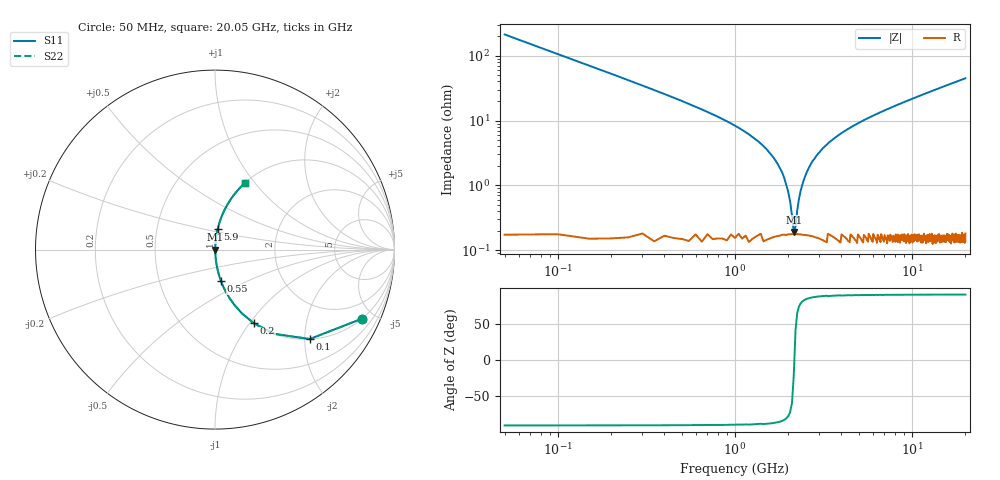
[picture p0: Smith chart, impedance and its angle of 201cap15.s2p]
! AVX Thin Film Operation		Date: May 2007
! Description: Accu-P® Series, Thin Film, SMD, RF Capacitor
! Part Number: 0201ZK150FBS
! 50 MHz  -  20.05 GHz
! Serial Measurements
# MHZ S MA R 50
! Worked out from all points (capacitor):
!   401 points, 50 MHz to 20.05 GHz, reference 50 ohm
!   read as one part in series: C = 15 pF near 150 MHz
!   lowest |Z| = 192 mohm at 2.15 GHz (marker M1)
!   series resonance near 2.166 GHz, so ESL is about 360 pH
!   S11 on the Smith chart (normalised r, x): 50 MHz: 1.01, -4.24; 100 MHz: 1.00, -2.12; 200 MHz: 1.00, -1.05; 550 MHz: 1.00, -0.36; 5.9 GHz: 1.00, +0.23; 20.05 GHz: 1.00, +0.90
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50  0.904 -25.2  0.426 64.7  0.426 64.7  0.904 -25.2
100  0.726 -43.3  0.686 46.6  0.686 46.6  0.726 -43.3
200  0.465 -62.1  0.884 27.7  0.884 27.7  0.465 -62.1
350  0.283 -73.3  0.958 16.4  0.958 16.4  0.283 -73.3
550  0.177 -79.3  0.983 10.2  0.983 10.2  0.177 -79.3
1400  0.044 -85.5  0.997 2.5  0.997 2.5  0.044 -85.5
1750  0.021 -84.6  0.998 1.2  0.998 1.2  0.021 -84.6
1950  0.01 -80.9  0.998 0.6  0.998 0.6  0.01 -80.9
2100  0.003393 -62.7  0.998 0.2  0.998 0.2  0.003393 -62.7
2150  0.001706 -24.8  0.998 0.0  0.998 0.0  0.001706 -24.8
2250  0.004039 67.3  0.998 -0.2  0.998 -0.2  0.004039 67.3
2350  0.008141 78.6  0.998 -0.5  0.998 -0.5  0.008141 78.6
2450  0.012 82.0  0.998 -0.7  0.998 -0.7  0.012 82.0
2650  0.02 84.4  0.998 -1.1  0.998 -1.1  0.02 84.4
3400  0.046 85.4  0.997 -2.6  0.997 -2.6  0.046 85.4
4450  0.076 84.5  0.996 -4.4  0.996 -4.4  0.076 84.5
5900  0.115 82.7  0.992 -6.6  0.992 -6.6  0.115 82.7
6750  0.135 81.6  0.989 -7.8  0.989 -7.8  0.135 81.6
10050  0.212 77.4  0.976 -12.2  0.976 -12.2  0.212 77.4
13400  0.283 73.3  0.958 -16.4  0.958 -16.4  0.283 73.3
16750  0.349 69.4  0.936 -20.4  0.936 -20.4  0.349 69.4
20050  0.408 65.7  0.911 -24.1  0.911 -24.1  0.408 65.7
